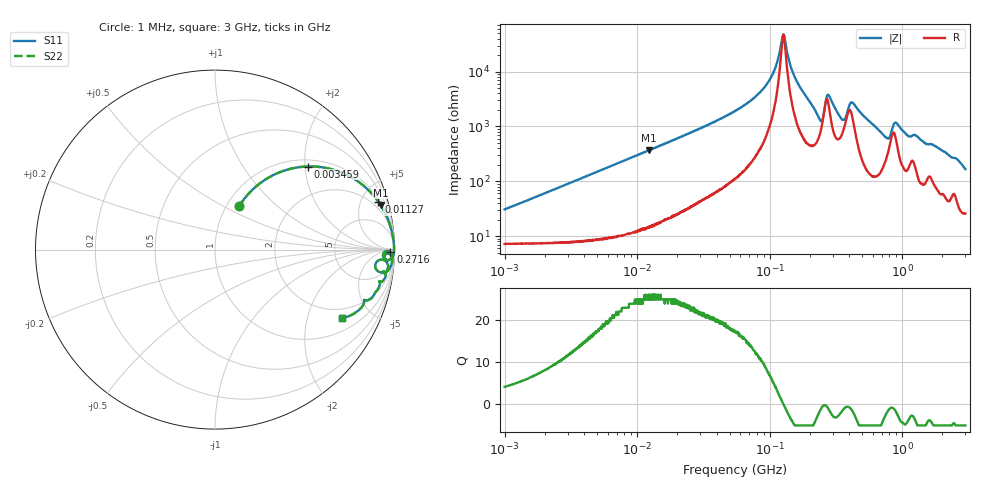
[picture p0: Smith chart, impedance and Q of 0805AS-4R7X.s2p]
!s-Parameter Generated by FASTRON Sdn. Bhd.
!FASTRON P/N : 0805AS-4R7X
!Keysight Technologies: E4991B_MY54100416_A.01.15
!Date: Mon Jun 15 12:59:25 2026
!Version  :Rev01  Mon Jun 15 12:59:25 2026
!Data & Calibration Information:
!Freq  S11  S21  S12  S22
!PortZ  Port1:50+j0  Port2:50+j0
!When reading reference impedance value at option line is always used.
! Remarks : This data is being provided solely for informational purposes.
# Hz S dB R 50
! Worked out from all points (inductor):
!   1601 points, 1 MHz to 3 GHz, reference 50 ohm
!   read as one part in series: L = 4.75 uH near 1.041 MHz
!   highest Q = 25.9 at 12.27 MHz (marker M1), where L = 4.76 uH
!   self-resonance near 127 MHz
!   S11 on the Smith chart (normalised r, x): 1 MHz: 1.14, +0.60; 3.459 MHz: 1.16, +2.06; 11.27 MHz: 1.28, +6.75; 271.6 MHz: 64, -37; 3 GHz: 1.51, -3.29
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1000000  -11.20 60.9  -0.93 -15.6  -0.93 -15.6  -11.20 60.9
3459026  -3.19 41.9  -3.48 -43.7  -3.48 -43.7  -3.19 41.9
3804036  -2.78 39.6  -3.90 -46.4  -3.90 -46.4  -2.78 39.6
1.126754e7  -0.46 16.3  -11.00 -71.4  -11.00 -71.4  -0.46 16.3
1.2268e7  -0.40 15.1  -11.70 -72.7  -11.70 -72.7  -0.40 15.1
1.447069e7  -0.30 12.9  -13.00 -74.9  -13.00 -74.9  -0.30 12.9
5.504702e7  -0.04 3.0  -25.70 -83.7  -25.70 -83.7  -0.04 3.0
9.593103e7  -0.02 0.9  -35.70 -81.9  -35.70 -81.9  -0.02 0.9
1.098084e8  -0.02 0.5  -41.20 -76.6  -41.20 -76.6  -0.02 0.5
1.269575e8  -0.02 0.0  -53.60 -3.5  -53.60 -3.5  -0.02 0.0
1.535465e8  -0.02 -0.7  -38.40 77.8  -38.40 77.8  -0.02 -0.7
2.083556e8  -0.07 -2.3  -27.90 77.5  -27.90 77.5  -0.07 -2.3
2.445387e8  -0.50 -3.0  -22.40 41.2  -22.40 41.2  -0.50 -3.0
2.716345e8  -0.20 -0.8  -31.50 29.8  -31.50 29.8  -0.20 -0.8
2.827291e8  -0.14 -1.3  -31.10 54.7  -31.10 54.7  -0.14 -1.3
3.523638e8  -0.36 -3.4  -22.90 53.8  -22.90 53.8  -0.36 -3.4
4.219165e8  -0.17 -1.8  -28.90 56.3  -28.90 56.3  -0.17 -1.8
7.925923e8  -0.90 -6.7  -16.60 44.9  -16.60 44.9  -0.90 -6.7
9.0272e8  -0.37 -4.2  -21.70 57.8  -21.70 57.8  -0.37 -4.2
1.10276e9  -0.39 -7.9  -17.00 68.1  -17.00 68.1  -0.39 -7.9
1.912199e9  -0.59 -13.7  -12.40 67.4  -12.40 67.4  -0.59 -13.7
3e9  -1.89 -28.5  -6.33 52.6  -6.33 52.6  -1.89 -28.5
